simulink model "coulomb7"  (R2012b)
settings: Solver=ode2  StartTime=0.0  StopTime=100  FixedStep=0.001  MaxStep=0.001  RelTol=1e-3
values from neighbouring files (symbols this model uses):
  c = 2200    [coulomb_1.m]    (also in coulomb_10.m = 0.1; coulomb_11.m = 0; coulomb_2.m; coulomb_3.m)
  FG = 500    [coulomb_1.m]    (also in coulomb_10.m = 10; coulomb_11.m = 10; coulomb_2.m; coulomb_3.m)
  k = 10    [coulomb_10.m]    (also in coulomb_11.m; diff_filter_1.m = 250; diff_filter_2.m = 250; dry_friction_1.m = 2200)
  m = 400    [coulomb_1.m]    (also in coulomb_10.m = 10; coulomb_11.m = 10; coulomb_2.m; coulomb_3.m)

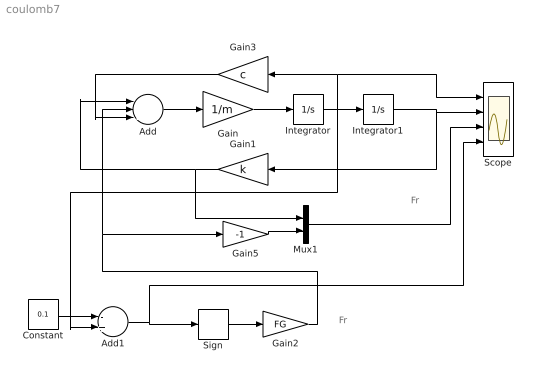
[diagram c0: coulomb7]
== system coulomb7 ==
  note: Fr
  note: Fr
  Add : Sum  Inputs=---
  Add1 : Sum  Inputs=-+
  Constant : Constant  Value=0.1
  Gain : Gain  Gain=1/m
  Gain1 : Gain  Gain=k
  Gain2 : Gain  Gain=FG
  Gain3 : Gain  Gain=c
  Gain5 : Gain  Gain=-1
  Integrator : Integrator
  Integrator1 : Integrator
  Mux1 : Mux  Inputs=2
  Scope : Scope  NumInputPorts=4
  Sign : Signum
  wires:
  Add/1 -> Gain/1
  Gain/1 -> Integrator/1
  Integrator1/1 -> Gain1/1, Scope/2
  Constant/1 -> Add1/1
  Integrator/1 -> Add1/2, Integrator1/1, Scope/1, Gain3/1
  Gain3/1 -> Add/3
  Gain1/1 -> Mux1/1, Add/1
  Mux1/1 -> Scope/3
  Add1/1 -> Sign/1, Scope/4
  Gain5/1 -> Mux1/2
  Sign/1 -> Gain2/1
  Gain2/1 -> Gain5/1, Add/2
